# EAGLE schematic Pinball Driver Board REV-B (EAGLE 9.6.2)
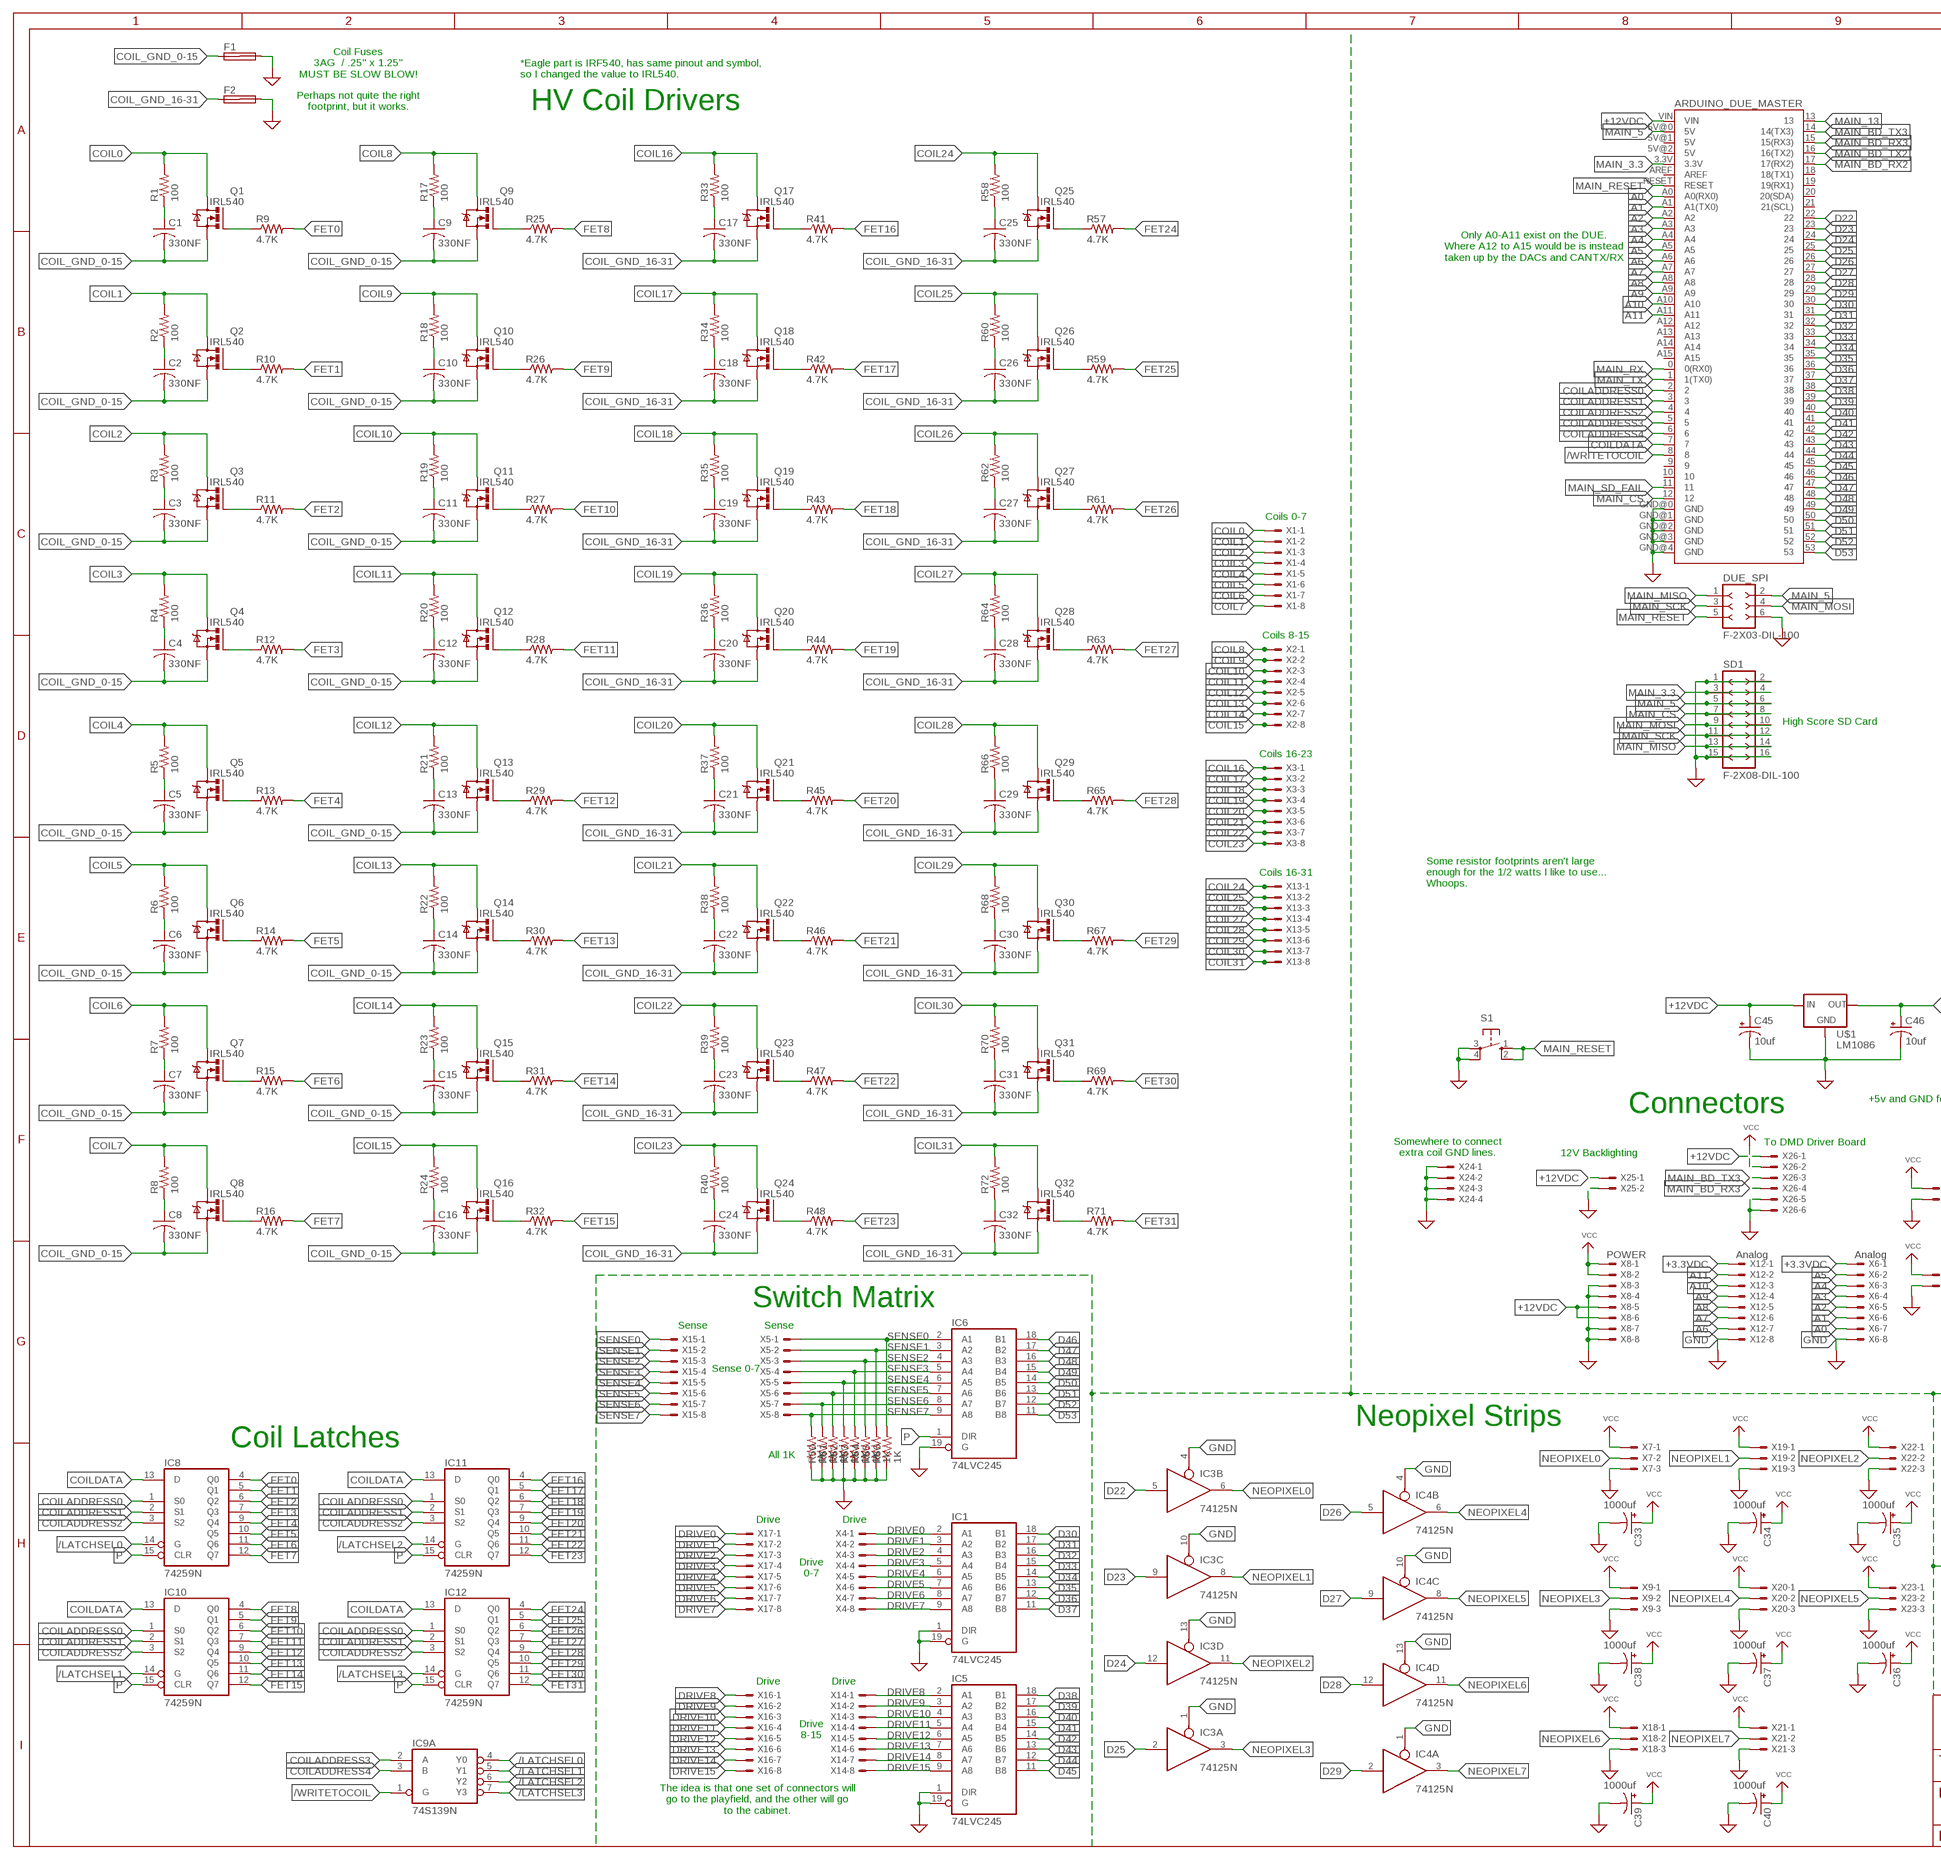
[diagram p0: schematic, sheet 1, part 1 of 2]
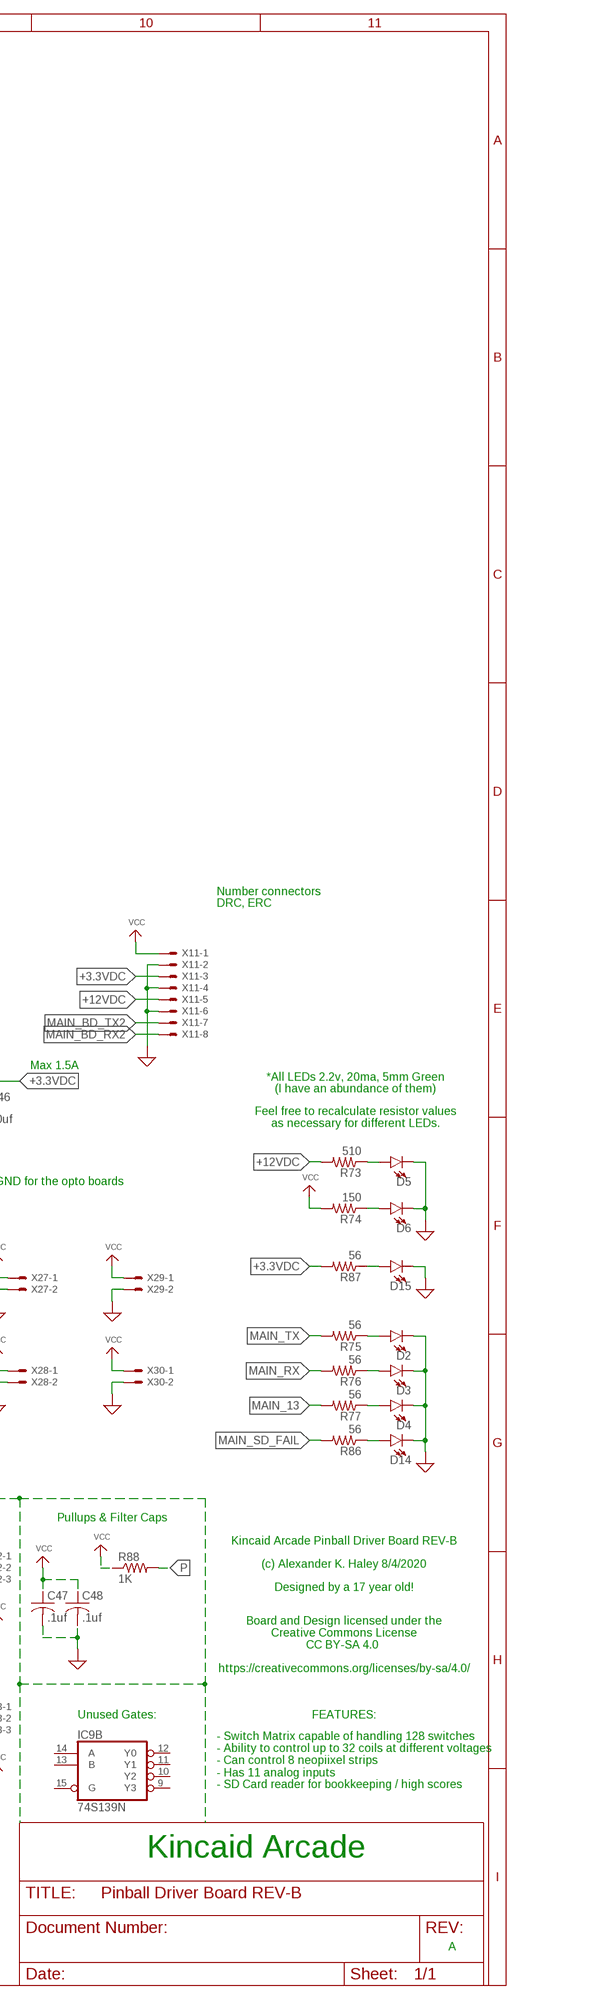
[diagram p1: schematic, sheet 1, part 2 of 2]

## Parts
ARDUINO_DUE_MASTER  ARDUINO_MEGA_R3FULL  [ARDUINO_MEGA]
C1  330NF  C-US150-054X183  [C150-054X183]
C2  330NF  C-US150-054X183  [C150-054X183]
C3  330NF  C-US150-054X183  [C150-054X183]
C4  330NF  C-US150-054X183  [C150-054X183]
C5  330NF  C-US150-054X183  [C150-054X183]
C6  330NF  C-US150-054X183  [C150-054X183]
C7  330NF  C-US150-054X183  [C150-054X183]
C8  330NF  C-US150-054X183  [C150-054X183]
C9  330NF  C-US150-054X183  [C150-054X183]
C10  330NF  C-US150-054X183  [C150-054X183]
C11  330NF  C-US150-054X183  [C150-054X183]
C12  330NF  C-US150-054X183  [C150-054X183]
C13  330NF  C-US150-054X183  [C150-054X183]
C14  330NF  C-US150-054X183  [C150-054X183]
C15  330NF  C-US150-054X183  [C150-054X183]
C16  330NF  C-US150-054X183  [C150-054X183]
C17  330NF  C-US150-054X183  [C150-054X183]
C18  330NF  C-US150-054X183  [C150-054X183]
C19  330NF  C-US150-054X183  [C150-054X183]
C20  330NF  C-US150-054X183  [C150-054X183]
C21  330NF  C-US150-054X183  [C150-054X183]
C22  330NF  C-US150-054X183  [C150-054X183]
C23  330NF  C-US150-054X183  [C150-054X183]
C24  330NF  C-US150-054X183  [C150-054X183]
C25  330NF  C-US150-054X183  [C150-054X183]
C26  330NF  C-US150-054X183  [C150-054X183]
C27  330NF  C-US150-054X183  [C150-054X183]
C28  330NF  C-US150-054X183  [C150-054X183]
C29  330NF  C-US150-054X183  [C150-054X183]
C30  330NF  C-US150-054X183  [C150-054X183]
C31  330NF  C-US150-054X183  [C150-054X183]
C32  330NF  C-US150-054X183  [C150-054X183]
C33  1000uf  CPOL-USB45181B  [B45181B]
C34  1000uf  CPOL-USB45181B  [B45181B]
C35  1000uf  CPOL-USB45181B  [B45181B]
C36  1000uf  CPOL-USB45181B  [B45181B]
C37  1000uf  CPOL-USB45181B  [B45181B]
C38  1000uf  CPOL-USB45181B  [B45181B]
C39  1000uf  CPOL-USB45181B  [B45181B]
C40  1000uf  CPOL-USB45181B  [B45181B]
C45  10uf  CPOL-USB45181A  [B45181A]
C46  10uf  CPOL-USB45181A  [B45181A]
C47  .1uf  C-US050-025X075  [C050-025X075]
C48  .1uf  C-US050-025X075  [C050-025X075]
D2  LED5MM-KIT  [LED_5MM-KIT]
D3  LED5MM-KIT  [LED_5MM-KIT]
D4  LED5MM-KIT  [LED_5MM-KIT]
D5  LED5MM-KIT  [LED_5MM-KIT]
D6  LED5MM-KIT  [LED_5MM-KIT]
D14  LED5MM-KIT  [LED_5MM-KIT]
D15  LED5MM-KIT  [LED_5MM-KIT]
DUE_SPI  F-2X03-DIL-100  [DIL-100-2X03]
F1  SH32  [SH32]
F2  SH32  [SH32]
IC1  74LVC245  74LS245N  [DIL20]
IC3  74125N  [DIL14]
IC4  74125N  [DIL14]
IC5  74LVC245  74LS245N  [DIL20]
IC6  74LVC245  74LS245N  [DIL20]
IC8  74259N  [DIL16]
IC9  74S139N  [DIL16]
IC10  74259N  [DIL16]
IC11  74259N  [DIL16]
IC12  74259N  [DIL16]
Q1  IRL540  IRF540  [TO220BV]
Q2  IRL540  IRF540  [TO220BV]
Q3  IRL540  IRF540  [TO220BV]
Q4  IRL540  IRF540  [TO220BV]
Q5  IRL540  IRF540  [TO220BV]
Q6  IRL540  IRF540  [TO220BV]
Q7  IRL540  IRF540  [TO220BV]
Q8  IRL540  IRF540  [TO220BV]
Q9  IRL540  IRF540  [TO220BV]
Q10  IRL540  IRF540  [TO220BV]
Q11  IRL540  IRF540  [TO220BV]
Q12  IRL540  IRF540  [TO220BV]
Q13  IRL540  IRF540  [TO220BV]
Q14  IRL540  IRF540  [TO220BV]
Q15  IRL540  IRF540  [TO220BV]
Q16  IRL540  IRF540  [TO220BV]
Q17  IRL540  IRF540  [TO220BV]
Q18  IRL540  IRF540  [TO220BV]
Q19  IRL540  IRF540  [TO220BV]
Q20  IRL540  IRF540  [TO220BV]
Q21  IRL540  IRF540  [TO220BV]
Q22  IRL540  IRF540  [TO220BV]
Q23  IRL540  IRF540  [TO220BV]
Q24  IRL540  IRF540  [TO220BV]
Q25  IRL540  IRF540  [TO220BV]
Q26  IRL540  IRF540  [TO220BV]
Q27  IRL540  IRF540  [TO220BV]
Q28  IRL540  IRF540  [TO220BV]
Q29  IRL540  IRF540  [TO220BV]
Q30  IRL540  IRF540  [TO220BV]
Q31  IRL540  IRF540  [TO220BV]
Q32  IRL540  IRF540  [TO220BV]
R1  100  R-US_0207/15  [0207/15]
R2  100  R-US_0207/15  [0207/15]
R3  100  R-US_0207/15  [0207/15]
R4  100  R-US_0207/15  [0207/15]
R5  100  R-US_0207/15  [0207/15]
R6  100  R-US_0207/15  [0207/15]
R7  100  R-US_0207/15  [0207/15]
R8  100  R-US_0207/15  [0207/15]
R9  4.7K  R-US_0207/10  [0207/10]
R10  4.7K  R-US_0207/10  [0207/10]
R11  4.7K  R-US_0207/10  [0207/10]
R12  4.7K  R-US_0207/10  [0207/10]
R13  4.7K  R-US_0207/10  [0207/10]
R14  4.7K  R-US_0207/10  [0207/10]
R15  4.7K  R-US_0207/10  [0207/10]
R16  4.7K  R-US_0207/10  [0207/10]
R17  100  R-US_0207/15  [0207/15]
R18  100  R-US_0207/15  [0207/15]
R19  100  R-US_0207/15  [0207/15]
R20  100  R-US_0207/15  [0207/15]
R21  100  R-US_0207/15  [0207/15]
R22  100  R-US_0207/15  [0207/15]
R23  100  R-US_0207/15  [0207/15]
R24  100  R-US_0207/15  [0207/15]
R25  4.7K  R-US_0207/10  [0207/10]
R26  4.7K  R-US_0207/10  [0207/10]
R27  4.7K  R-US_0207/10  [0207/10]
R28  4.7K  R-US_0207/10  [0207/10]
R29  4.7K  R-US_0207/10  [0207/10]
R30  4.7K  R-US_0207/10  [0207/10]
R31  4.7K  R-US_0207/10  [0207/10]
R32  4.7K  R-US_0207/10  [0207/10]
R33  100  R-US_0207/15  [0207/15]
R34  100  R-US_0207/15  [0207/15]
R35  100  R-US_0207/15  [0207/15]
R36  100  R-US_0207/15  [0207/15]
R37  100  R-US_0207/15  [0207/15]
R38  100  R-US_0207/15  [0207/15]
R39  100  R-US_0207/15  [0207/15]
R40  100  R-US_0207/15  [0207/15]
R41  4.7K  R-US_0207/10  [0207/10]
R42  4.7K  R-US_0207/10  [0207/10]
R43  4.7K  R-US_0207/10  [0207/10]
R44  4.7K  R-US_0207/10  [0207/10]
R45  4.7K  R-US_0207/10  [0207/10]
R46  4.7K  R-US_0207/10  [0207/10]
R47  4.7K  R-US_0207/10  [0207/10]
R48  4.7K  R-US_0207/10  [0207/10]
R49  1K  R-US_0204/7  [0204/7]
R50  1K  R-US_0204/7  [0204/7]
R51  1K  R-US_0204/7  [0204/7]
R52  1K  R-US_0204/7  [0204/7]
R53  1K  R-US_0204/7  [0204/7]
R54  1K  R-US_0204/7  [0204/7]
R55  1K  R-US_0204/7  [0204/7]
R56  1K  R-US_0204/7  [0204/7]
R57  4.7K  R-US_0207/10  [0207/10]
R58  100  R-US_0207/15  [0207/15]
R59  4.7K  R-US_0207/10  [0207/10]
R60  100  R-US_0207/15  [0207/15]
R61  4.7K  R-US_0207/10  [0207/10]
R62  100  R-US_0207/15  [0207/15]
R63  4.7K  R-US_0207/10  [0207/10]
R64  100  R-US_0207/15  [0207/15]
R65  4.7K  R-US_0207/10  [0207/10]
R66  100  R-US_0207/15  [0207/15]
R67  4.7K  R-US_0207/10  [0207/10]
R68  100  R-US_0207/15  [0207/15]
R69  4.7K  R-US_0207/10  [0207/10]
R70  100  R-US_0207/15  [0207/15]
R71  4.7K  R-US_0207/10  [0207/10]
R72  100  R-US_0207/15  [0207/15]
R73  510  R-US_0207/7  [0207/7]
R74  150  R-US_0207/7  [0207/7]
R75  56  R-US_0207/7  [0207/7]
R76  56  R-US_0207/7  [0207/7]
R77  56  R-US_0207/7  [0207/7]
R86  56  R-US_0207/7  [0207/7]
R87  56  R-US_0207/7  [0207/7]
R88  1K  R-US_0207/7  [0207/7]
S1  10-XX  [B3F-10XX]
SD1  F-2X08-DIL-100  [DIL-100-2X08]
U$1  LM1086  [78XXL]
X1  Coils 0-7  KK-156-8  [KK-156-8]
X2  Coils 8-15  KK-156-8  [KK-156-8]
X3  Coils 16-23  KK-156-8  [KK-156-8]
X4  Columns 0-7  KK-156-8  [KK-156-8]
X5  Rows 0-7  KK-156-8  [KK-156-8]
X6  Analog  KK-156-8  [KK-156-8]
X7  KK-156-3  [KK-156-3]
X8  POWER  KK-156-8  [KK-156-8]
X9  KK-156-3  [KK-156-3]
X11  KK-156-8  [KK-156-8]
X12  Analog  KK-156-8  [KK-156-8]
X13  Coils 16-31  KK-156-8  [KK-156-8]
X14  Columns 8-15  KK-156-8  [KK-156-8]
X15  Rows 0-7  KK-156-8  [KK-156-8]
X16  Columns 8-15  KK-156-8  [KK-156-8]
X17  Columns 0-7  KK-156-8  [KK-156-8]
X18  KK-156-3  [KK-156-3]
X19  KK-156-3  [KK-156-3]
X20  KK-156-3  [KK-156-3]
X21  KK-156-3  [KK-156-3]
X22  KK-156-3  [KK-156-3]
X23  KK-156-3  [KK-156-3]
X24  KK-156-4  [KK-156-4]
X25  KK-156-2  [KK-156-2]
X26  KK-156-6  [KK-156-6]
X27  KK-156-2  [KK-156-2]
X28  KK-156-2  [KK-156-2]
X29  KK-156-2  [KK-156-2]
X30  KK-156-2  [KK-156-2]

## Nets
+3.3VDC: C46.+ R87.2 U$1.OUT X6.1 X11.3 X12.1
+12VDC: ARDUINO_DUE_MASTER.VIN C45.+ R73.2 U$1.IN X8.5 X8.6 X11.5 X25.1 X26.1
/LATCHSEL0: IC8.14(G) IC9.4(A:Y0)
/LATCHSEL1: IC9.5(A:Y1) IC10.14(G)
/LATCHSEL2: IC9.6(A:Y2) IC11.14(G)
/LATCHSEL3: IC9.7(A:Y3) IC12.14(G)
/WRITETOCOIL: ARDUINO_DUE_MASTER.8 IC9.1(A:G)
A0: ARDUINO_DUE_MASTER.A0(A0(RX0)) X6.7
A1: ARDUINO_DUE_MASTER.A1(A1(TX0)) X6.6
A2: ARDUINO_DUE_MASTER.A2 X6.5
A3: ARDUINO_DUE_MASTER.A3 X6.4
A4: ARDUINO_DUE_MASTER.A4 X6.3
A5: ARDUINO_DUE_MASTER.A5 X6.2
A6: ARDUINO_DUE_MASTER.A6 X12.7
A7: ARDUINO_DUE_MASTER.A7 X12.6
A8: ARDUINO_DUE_MASTER.A8 X12.5
A9: ARDUINO_DUE_MASTER.A9 X12.4
A10: ARDUINO_DUE_MASTER.A10 X12.3
A11: ARDUINO_DUE_MASTER.A11 X12.2
COIL0: Q1.D R1.2 X1.1
COIL1: Q2.D R2.2 X1.2
COIL2: Q3.D R3.2 X1.3
COIL3: Q4.D R4.2 X1.4
COIL4: Q5.D R5.2 X1.5
COIL5: Q6.D R6.2 X1.6
COIL6: Q7.D R7.2 X1.7
COIL7: Q8.D R8.2 X1.8
COIL8: Q9.D R17.2 X2.1
COIL9: Q10.D R18.2 X2.2
COIL10: Q11.D R19.2 X2.3
COIL11: Q12.D R20.2 X2.4
COIL12: Q13.D R21.2 X2.5
COIL13: Q14.D R22.2 X2.6
COIL14: Q15.D R23.2 X2.7
COIL15: Q16.D R24.2 X2.8
COIL16: Q17.D R33.2 X3.1
COIL17: Q18.D R34.2 X3.2
COIL18: Q19.D R35.2 X3.3
COIL19: Q20.D R36.2 X3.4
COIL20: Q21.D R37.2 X3.5
COIL21: Q22.D R38.2 X3.6
COIL22: Q23.D R39.2 X3.7
COIL23: Q24.D R40.2 X3.8
COIL24: Q25.D R58.2 X13.1
COIL25: Q26.D R60.2 X13.2
COIL26: Q27.D R62.2 X13.3
COIL27: Q28.D R64.2 X13.4
COIL28: Q29.D R66.2 X13.5
COIL29: Q30.D R68.2 X13.6
COIL30: Q31.D R70.2 X13.7
COIL31: Q32.D R72.2 X13.8
COIL_GND_0-15: C1.2 C2.2 C3.2 C4.2 C5.2 C6.2 C7.2 C8.2 C9.2 C10.2 C11.2 C12.2 C13.2 C14.2 C15.2 C16.2 F1.1A Q1.S Q2.S Q3.S Q4.S Q5.S Q6.S Q7.S Q8.S Q9.S Q10.S Q11.S Q12.S Q13.S Q14.S Q15.S Q16.S
COIL_GND_16-31: C17.2 C18.2 C19.2 C20.2 C21.2 C22.2 C23.2 C24.2 C25.2 C26.2 C27.2 C28.2 C29.2 C30.2 C31.2 C32.2 F2.1A Q17.S Q18.S Q19.S Q20.S Q21.S Q22.S Q23.S Q24.S Q25.S Q26.S Q27.S Q28.S Q29.S Q30.S Q31.S Q32.S
COILADDRESS0: ARDUINO_DUE_MASTER.2 IC8.1(S0) IC10.1(S0) IC11.1(S0) IC12.1(S0)
COILADDRESS1: ARDUINO_DUE_MASTER.3 IC8.2(S1) IC10.2(S1) IC11.2(S1) IC12.2(S1)
COILADDRESS2: ARDUINO_DUE_MASTER.4 IC8.3(S2) IC10.3(S2) IC11.3(S2) IC12.3(S2)
COILADDRESS3: ARDUINO_DUE_MASTER.5 IC9.2(A:A)
COILADDRESS4: ARDUINO_DUE_MASTER.6 IC9.3(A:B)
COILDATA: ARDUINO_DUE_MASTER.7 IC8.13(D) IC10.13(D) IC11.13(D) IC12.13(D)
D22: ARDUINO_DUE_MASTER.22 IC3.5(B:I)
D23: ARDUINO_DUE_MASTER.23 IC3.9(C:I)
D24: ARDUINO_DUE_MASTER.24 IC3.12(D:I)
D25: ARDUINO_DUE_MASTER.25 IC3.2(A:I)
D26: ARDUINO_DUE_MASTER.26 IC4.5(B:I)
D27: ARDUINO_DUE_MASTER.27 IC4.9(C:I)
D28: ARDUINO_DUE_MASTER.28 IC4.12(D:I)
D29: ARDUINO_DUE_MASTER.29 IC4.2(A:I)
D30: ARDUINO_DUE_MASTER.30 IC1.18(B1)
D31: ARDUINO_DUE_MASTER.31 IC1.17(B2)
D32: ARDUINO_DUE_MASTER.32 IC1.16(B3)
D33: ARDUINO_DUE_MASTER.33 IC1.15(B4)
D34: ARDUINO_DUE_MASTER.34 IC1.14(B5)
D35: ARDUINO_DUE_MASTER.35 IC1.13(B6)
D36: ARDUINO_DUE_MASTER.36 IC1.12(B7)
D37: ARDUINO_DUE_MASTER.37 IC1.11(B8)
D38: ARDUINO_DUE_MASTER.38 IC5.18(B1)
D39: ARDUINO_DUE_MASTER.39 IC5.17(B2)
D40: ARDUINO_DUE_MASTER.40 IC5.16(B3)
D41: ARDUINO_DUE_MASTER.41 IC5.15(B4)
D42: ARDUINO_DUE_MASTER.42 IC5.14(B5)
D43: ARDUINO_DUE_MASTER.43 IC5.13(B6)
D44: ARDUINO_DUE_MASTER.44 IC5.12(B7)
D45: ARDUINO_DUE_MASTER.45 IC5.11(B8)
D46: ARDUINO_DUE_MASTER.46 IC6.18(B1)
D47: ARDUINO_DUE_MASTER.47 IC6.17(B2)
D48: ARDUINO_DUE_MASTER.48 IC6.16(B3)
D49: ARDUINO_DUE_MASTER.49 IC6.15(B4)
D50: ARDUINO_DUE_MASTER.50 IC6.14(B5)
D51: ARDUINO_DUE_MASTER.51 IC6.13(B6)
D52: ARDUINO_DUE_MASTER.52 IC6.12(B7)
D53: ARDUINO_DUE_MASTER.53 IC6.11(B8)
DRIVE0: IC1.2(A1) X4.1 X17.1
DRIVE1: IC1.3(A2) X4.2 X17.2
DRIVE2: IC1.4(A3) X4.3 X17.3
DRIVE3: IC1.5(A4) X4.4 X17.4
DRIVE4: IC1.6(A5) X4.5 X17.5
DRIVE5: IC1.7(A6) X4.6 X17.6
DRIVE6: IC1.8(A7) X4.7 X17.7
DRIVE7: IC1.9(A8) X4.8 X17.8
DRIVE8: IC5.2(A1) X14.1 X16.1
DRIVE9: IC5.3(A2) X14.2 X16.2
DRIVE10: IC5.4(A3) X14.3 X16.3
DRIVE11: IC5.5(A4) X14.4 X16.4
DRIVE12: IC5.6(A5) X14.5 X16.5
DRIVE13: IC5.7(A6) X14.6 X16.6
DRIVE14: IC5.8(A7) X14.7 X16.7
DRIVE15: IC5.9(A8) X14.8 X16.8
FET0: IC8.4(Q0) R9.2
FET1: IC8.5(Q1) R10.2
FET2: IC8.6(Q2) R11.2
FET3: IC8.7(Q3) R12.2
FET4: IC8.9(Q4) R13.2
FET5: IC8.10(Q5) R14.2
FET6: IC8.11(Q6) R15.2
FET7: IC8.12(Q7) R16.2
FET8: IC10.4(Q0) R25.2
FET9: IC10.5(Q1) R26.2
FET10: IC10.6(Q2) R27.2
FET11: IC10.7(Q3) R28.2
FET12: IC10.9(Q4) R29.2
FET13: IC10.10(Q5) R30.2
FET14: IC10.11(Q6) R31.2
FET15: IC10.12(Q7) R32.2
FET16: IC11.4(Q0) R41.2
FET17: IC11.5(Q1) R42.2
FET18: IC11.6(Q2) R43.2
FET19: IC11.7(Q3) R44.2
FET20: IC11.9(Q4) R45.2
FET21: IC11.10(Q5) R46.2
FET22: IC11.11(Q6) R47.2
FET23: IC11.12(Q7) R48.2
FET24: IC12.4(Q0) R57.2
FET25: IC12.5(Q1) R59.2
FET26: IC12.6(Q2) R61.2
FET27: IC12.7(Q3) R63.2
FET28: IC12.9(Q4) R65.2
FET29: IC12.10(Q5) R67.2
FET30: IC12.11(Q6) R69.2
FET31: IC12.12(Q7) R71.2
GND: ARDUINO_DUE_MASTER.GND@0(GND) ARDUINO_DUE_MASTER.GND@1(GND) ARDUINO_DUE_MASTER.GND@2(GND) ARDUINO_DUE_MASTER.GND@3(GND) ARDUINO_DUE_MASTER.GND@4(GND) C33.- C34.- C35.- C36.- C37.- C38.- C39.- C40.- C45.- C46.- C47.2 C48.2 D2.K(C) D3.K(C) D4.K(C) D5.K(C) D6.K(C) D14.K(C) D15.K(C) DUE_SPI.6 F1.2A F2.2A IC1.1(DIR) IC1.19(G) IC3.1(A:OE) IC3.4(B:OE) IC3.10(C:OE) IC3.13(D:OE) IC4.1(A:OE) IC4.4(B:OE) IC4.10(C:OE) IC4.13(D:OE) IC5.1(DIR) IC5.19(G) IC6.19(G) R49.1 R50.1 R51.1 R52.1 R53.1 R54.1 R55.1 R56.1 S1.3(P) S1.4(P1) SD1.1 SD1.2 SD1.15 SD1.16 U$1.GND X6.8 X7.3 X8.3 X8.4 X8.7 X8.8 X9.3 X11.2 X11.4 X11.6 X12.8 X18.3 X19.3 X20.3 X21.3 X22.3 X23.3 X24.1 X24.2 X24.3 X24.4 X25.2 X26.5 X26.6 X27.2 X28.2 X29.2 X30.2 ; supply symbol labelled SUP
MAIN_3.3: ARDUINO_DUE_MASTER.3.3V SD1.3 SD1.4
MAIN_5: ARDUINO_DUE_MASTER.5V@0(5V) DUE_SPI.2 SD1.5 SD1.6
MAIN_13: ARDUINO_DUE_MASTER.13 R77.2
MAIN_BD_RX2: ARDUINO_DUE_MASTER.17(17(RX2)) X11.8
MAIN_BD_RX3: ARDUINO_DUE_MASTER.15(15(RX3)) X26.4
MAIN_BD_TX2: ARDUINO_DUE_MASTER.16(16(TX2)) X11.7
MAIN_BD_TX3: ARDUINO_DUE_MASTER.14(14(TX3)) X26.3
MAIN_CS: ARDUINO_DUE_MASTER.12 SD1.7 SD1.8
MAIN_MISO: DUE_SPI.1 SD1.13 SD1.14
MAIN_MOSI: DUE_SPI.4 SD1.9 SD1.10
MAIN_RESET: ARDUINO_DUE_MASTER.RESET DUE_SPI.5 S1.1(S) S1.2(S1)
MAIN_RX: ARDUINO_DUE_MASTER.0(0(RX0)) R76.2
MAIN_SCK: DUE_SPI.3 SD1.11 SD1.12
MAIN_SD_FAIL: ARDUINO_DUE_MASTER.11 R86.2
MAIN_TX: ARDUINO_DUE_MASTER.1(1(TX0)) R75.2
N$1: Q2.G R10.1
N$3: Q1.G R9.1
N$4: D14.A R86.1
N$5: C1.1 R1.1
N$6: C2.1 R2.1
N$7: Q3.G R11.1
N$8: D15.A R87.1
N$9: Q17.G R41.1
N$10: C3.1 R3.1
N$12: Q4.G R12.1
N$14: C4.1 R4.1
N$15: Q5.G R13.1
N$17: C5.1 R5.1
N$18: C17.1 R33.1
N$19: Q6.G R14.1
N$21: C6.1 R6.1
N$22: Q18.G R42.1
N$23: Q7.G R15.1
N$25: C7.1 R7.1
N$26: Q8.G R16.1
N$28: C8.1 R8.1
N$29: Q9.G R25.1
N$30: D2.A R75.1
N$31: D3.A R76.1
N$32: C9.1 R17.1
N$33: Q10.G R26.1
N$34: D4.A R77.1
N$35: C10.1 R18.1
N$36: Q11.G R27.1
N$38: C11.1 R19.1
N$39: Q12.G R28.1
N$41: C12.1 R20.1
N$42: Q13.G R29.1
N$44: C18.1 R34.1
N$45: C13.1 R21.1
N$46: Q14.G R30.1
N$48: C14.1 R22.1
N$49: Q15.G R31.1
N$51: C15.1 R23.1
N$52: Q16.G R32.1
N$53: D6.A R74.1
N$54: C16.1 R24.1
N$55: Q19.G R43.1
N$56: D5.A R73.1
N$57: C19.1 R35.1
N$58: Q20.G R44.1
N$60: C20.1 R36.1
N$61: Q21.G R45.1
N$63: C21.1 R37.1
N$64: Q22.G R46.1
N$66: C22.1 R38.1
N$67: Q23.G R47.1
N$69: C23.1 R39.1
N$70: Q24.G R48.1
N$72: C24.1 R40.1
N$73: Q25.G R57.1
N$74: C25.1 R58.1
N$75: Q26.G R59.1
N$76: C26.1 R60.1
N$77: Q27.G R61.1
N$78: C27.1 R62.1
N$79: Q28.G R63.1
N$80: C28.1 R64.1
N$81: Q29.G R65.1
N$82: C29.1 R66.1
N$83: Q30.G R67.1
N$84: C30.1 R68.1
N$85: Q31.G R69.1
N$86: C31.1 R70.1
N$87: Q32.G R71.1
N$88: C32.1 R72.1
NEOPIXEL0: IC3.6(B:O) X7.2
NEOPIXEL1: IC3.8(C:O) X19.2
NEOPIXEL2: IC3.11(D:O) X22.2
NEOPIXEL3: IC3.3(A:O) X9.2
NEOPIXEL4: IC4.6(B:O) X20.2
NEOPIXEL5: IC4.8(C:O) X23.2
NEOPIXEL6: IC4.11(D:O) X18.2
NEOPIXEL7: IC4.3(A:O) X21.2
P: IC6.1(DIR) IC8.15(CLR) IC10.15(CLR) IC11.15(CLR) IC12.15(CLR) R88.2
SENSE0: IC6.2(A1) R56.2 X5.1 X15.1
SENSE1: IC6.3(A2) R55.2 X5.2 X15.2
SENSE2: IC6.4(A3) R54.2 X5.3 X15.3
SENSE3: IC6.5(A4) R53.2 X5.4 X15.4
SENSE4: IC6.6(A5) R52.2 X5.5 X15.5
SENSE5: IC6.7(A6) R51.2 X5.6 X15.6
SENSE6: IC6.8(A7) R50.2 X5.7 X15.7
SENSE7: IC6.9(A8) R49.2 X5.8 X15.8
VCC: C33.+ C34.+ C35.+ C36.+ C37.+ C38.+ C39.+ C40.+ C47.1 C48.1 R74.2 R88.1 X7.1 X8.1 X8.2 X9.1 X11.1 X18.1 X19.1 X20.1 X21.1 X22.1 X23.1 X26.2 X27.1 X28.1 X29.1 X30.1
Unconnected: ARDUINO_DUE_MASTER.5V@1(5V) ARDUINO_DUE_MASTER.5V@2(5V) ARDUINO_DUE_MASTER.9 ARDUINO_DUE_MASTER.10 ARDUINO_DUE_MASTER.18(18(TX1)) ARDUINO_DUE_MASTER.19(19(RX1)) ARDUINO_DUE_MASTER.20(20(SDA)) ARDUINO_DUE_MASTER.21(21(SCL)) ARDUINO_DUE_MASTER.A12 ARDUINO_DUE_MASTER.A13 ARDUINO_DUE_MASTER.A14 ARDUINO_DUE_MASTER.A15 ARDUINO_DUE_MASTER.AREF F1.1B F1.2B F2.1B F2.2B IC9.9(B:Y3) IC9.10(B:Y2) IC9.11(B:Y1) IC9.12(B:Y0) IC9.13(B:B) IC9.14(B:A) IC9.15(B:G)

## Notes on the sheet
- Coil Fuses
  3AG  / .25" x 1.25"
  MUST BE SLOW BLOW!
- *Eagle part is IRF540, has same pinout and symbol,
  so I changed the value to IRL540.
- Perhaps not quite the right
  footprint, but it works.
- HV Coil Drivers
- Only A0-A11 exist on the DUE.
  Where A12 to A15 would be is instead
  taken up by the DACs and CANTX/RX
- Coils 0-7
- Coils 8-15
- High Score SD Card
- Coils 16-23
- Number connectors
- DRC, ERC
- Coils 16-31
- Some resistor footprints aren't large
  enough for the 1/2 watts I like to use...
- Whoops.
- Max 1.5A
- *All LEDs 2.2v, 20ma, 5mm Green
- (I have an abundance of them)
- Feel free to recalculate resistor values
  as necessary for different LEDs.
- +5v and GND for the opto boards
- Connectors
- To DMD Driver Board
- Somewhere to connect
  extra coil GND lines.
- 12V Backlighting
- Switch Matrix
- Sense | Sense
- Sense 0-7
- Pullups & Filter Caps
- Neopixel Strips
- Kincaid Arcade Pinball Driver Board REV-B
- Coil Latches
- All 1K | (c) Alexander K. Haley 8/4/2020
- Designed by a 17 year old!
- Drive | Drive
- Board and Design licensed under the
  Creative Commons License
  CC BY-SA 4.0
- https://creativecommons.org/licenses/by-sa/4.0/
- Drive
  0-7
- Unused Gates: | FEATURES:
- - Switch Matrix capable of handling 128 switches
  - Ability to control up to 32 coils at different voltages
  - Can control 8 neopiixel strips
  - Has 11 analog inputs
- - SD Card reader for bookkeeping / high scores
- Drive | Drive
- Kincaid Arcade
- Drive
  8-15
- The idea is that one set of connectors will
  go to the playfield, and the other will go
  to the cabinet.
- A

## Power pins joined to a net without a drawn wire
GND: IC1.10(GND) IC3.7(P:GND) IC4.7(P:GND) IC5.10(GND) IC6.10(GND) IC8.8(GND) IC9.8(P:GND) IC10.8(GND) IC11.8(GND) IC12.8(GND)
VCC: IC1.20(VCC) IC3.14(P:VCC) IC4.14(P:VCC) IC5.20(VCC) IC6.20(VCC) IC8.16(VCC) IC9.16(P:VCC) IC10.16(VCC) IC11.16(VCC) IC12.16(VCC)

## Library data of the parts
ARDUINO_DUE_MASTER = SparkFun-Boards:ARDUINO_MEGA_R3: Arduino Mega R3 ATmega2560 R3 compatible footprint. SparkFun Products: Arduino Mega 2560 R3
C1-C32 = resistor:C-US: CAPACITOR, American symbol
C33-C40 = rcl:CPOL-US: POLARIZED CAPACITOR, American symbol; SPICEPREFIX: C
C45 C46 = adafruit:CPOL-US: POLARIZED CAPACITOR, American symbol
C47 C48 = rcl:C-US: CAPACITOR, American symbol; SPICEPREFIX: C
D2-D6 D14 D15 = SparkFun-LED:LED: LED (Generic)
DUE_SPI = con-headers-jp:F-2X03-: FEMALE HEADER
F1 F2 = fuse:SH32: FUSE HOLDER 6 x 32 mm, SH contact, SHH3N Schukat, 102071 Wickmann (Buerklin); MPN: 10207101009; OC_FARNELL: 811786; OC_NEWARK: 76R6904
IC1 IC5 IC6 = 74xx-us:74*245: Octal BUS TRANSCEIVER, 3-state
IC3 IC4 = 74xx-us:74*125: Quad bus BUFFER, 3-state
IC8 IC10-IC12 = 74xx-us:74*259: 8-bit addressable LATCH
IC9 = 74xx-us:74*139: Dual 2-line to 4-line DECODER/DEMULTIPLEXER
Q1-Q32 = transistor-power:IRF540: HEXFET Power MOSFET
R1-R72 = resistor:R-US_: RESISTOR, American symbol
R73-R77 R86-R88 = rcl:R-US_: RESISTOR, American symbol; SPICEPREFIX: R
S1 = switch-omron:10-XX: OMRON SWITCH; MPN: B3F-1000; OC_FARNELL: 176432; OC_NEWARK: 36M3542
SD1 = con-headers-jp:F-2X08-: FEMALE HEADER
U$1 = OLD AND OBSOLETE ARCADE PARTS:LM1086
X1-X6 X8 X11-X17 = con-molex:KK-156-8: KK 156 HEADER Source: http://www.molex.com/pdm_docs/sd/026604100_sd.pdf; MF: MOLEX; OC_FARNELL: unknown; OC_NEWARK: unknown
X7 X9 X18-X23 = con-molex:KK-156-3: KK 156 HEADER Source: http://www.molex.com/pdm_docs/sd/026604100_sd.pdf; MF: MOLEX; OC_FARNELL: unknown; OC_NEWARK: unknown
X24 = con-molex:KK-156-4: KK 156 HEADER Source: http://www.molex.com/pdm_docs/sd/026604100_sd.pdf; MF: MOLEX; OC_FARNELL: unknown; OC_NEWARK: unknown
X25 X27-X30 = con-molex:KK-156-2: KK 156 HEADER; MF: MOLEX; OC_FARNELL: unknown; OC_NEWARK: unknown
X26 = con-molex:KK-156-6: KK 156 HEADER Source: http://www.molex.com/pdm_docs/sd/026604100_sd.pdf; MF: MOLEX; OC_FARNELL: unknown; OC_NEWARK: unknown

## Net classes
0 default: width 0.406 mm, clearance 0.406 mm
